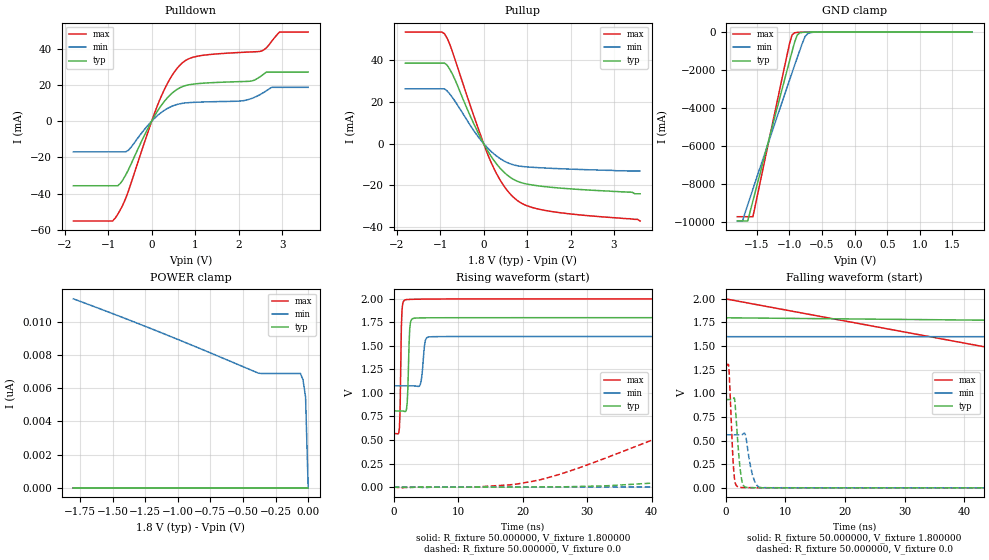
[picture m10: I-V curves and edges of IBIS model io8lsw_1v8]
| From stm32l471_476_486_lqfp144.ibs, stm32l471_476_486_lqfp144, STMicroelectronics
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|   Model io8lsw_1v8
[Model]  io8lsw_1v8
Model_type I/O
Polarity   Non-Inverting
Enable   Active-Low
Vinl =   0.540000V
Vinh =   1.260000V
Vmeas =  0.900000V
Cref =   100.000000nF
Rref =   1.000000k
Vref =   1.800000V
C_comp   3.002600pF   2.845500pF   3.023700pF
[Temperature Range]   25.000000   0.125000k   -40.000000
[Pullup Reference]   1.800000V   1.600000V   2.000000V
[Pulldown Reference]   0.0V   0.0V   0.0V
[POWER Clamp Reference]   1.800000V   1.600000V   2.000000V
[GND Clamp Reference]   0.0V   0.0V   0.0V
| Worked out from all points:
|   slope of the pulldown table from 0 to 0.27 V, typ, clamps not added: 26.4 ohm
|   slope of the pullup table from 0 to 0.27 V, typ, clamps not added: 30.1 ohm
|   GND clamp passes 1 mA (typ) near -0.58 V on its own axis
|   rising waveform, R_fixture 50.000000, V_fixture 1.800000: 20-80 % time 262ps typ, 404ps min, 194ps max; typ from 0.809 V to 1.8 V
|   rising waveform, R_fixture 50.000000, V_fixture 0.0: 20-80 % time 64.5ns typ, 115ns min, 35.9ns max; typ from 0 V to 0.934 V
|   falling waveform, R_fixture 50.000000, V_fixture 1.800000: 20-80 % time 75.9ns typ, 121ns min, 63ns max; typ from 1.8 V to 0.809 V
|   falling waveform, R_fixture 50.000000, V_fixture 0.0: 20-80 % time 713ps typ, 1.02ns min, 552ps max; typ from 0.934 V to 0 V
[Pulldown]
|Voltage   I(typ)   I(min)   I(max)
-1.8V     -35.64mA   -16.93mA   -55.1mA
-840mV    -35.64mA   -16.93mA   -53.52mA
-720mV    -34.31mA   -16.93mA   -48.86mA
-540mV    -27.04mA   -16.13mA   -38.89mA
240mV     9.303mA    5.14mA     14.78mA
480mV     15.67mA    8.374mA    25.64mA
720mV     19.18mA    9.883mA    32.46mA
1.08V     20.76mA    10.49mA    35.96mA
2.1V      21.86mA    11.27mA    37.98mA
2.52V     24.95mA    15.02mA    38.63mA
2.94V     27.08mA    18.65mA    49.17mA
3.6V      27.08mA    18.65mA    49.17mA
[Pullup]
|Voltage   I(typ)   I(min)   I(max)
-1.8V     38.39mA    26.12mA    53.23mA
-960mV    38.39mA    26.12mA    53.23mA
-900mV    38.39mA    26.12mA    52.4mA
-840mV    37.45mA    25.13mA    50.31mA
-720mV    33.22mA    22.05mA    44.01mA
-240mV    10.08mA    6.588mA    14.1mA
120mV     -4.38mA    -2.702mA   -6.45mA
420mV     -12.68mA   -7.723mA   -18.77mA
720mV     -17.48mA   -10.37mA   -26.28mA
1.02V     -19.45mA   -11.2mA    -29.89mA
1.44V     -20.66mA   -11.73mA   -32.03mA
3.6V      -24mA      -13.1mA    -37mA
[GND_clamp]
|Voltage   I(typ)   I(min)   I(max)
-1.8V     -9.93A     -9.932A    -9.707A
-1.72V    -9.93A     -9.932A    -9.707A
-1.64V    -9.93A     -9.083A    -9.707A
-1.56V    -8.876A    -8.251A    -9.707A
-1V       -1.54A     -2.541A    -631mA
-960mV    -1.028A    -2.139A    -153.7mA
-920mV    -527mA     -1.74A     -39.12mA
-880mV    -155.6mA   -1.344A    -18.01mA
-840mV    -45.32mA   -953mA     -12.68mA
-760mV    -8.418mA   -235mA     -7.62mA
-680mV    -3.44mA    -33.01mA   -3.865mA
1.8V      0A         0A         0A
[POWER_clamp]
|Voltage   I(typ)   I(min)   I(max)
-1.8V     0A         11.37nA    0A
-1.14V    0A         9.374nA    0A
-380mV    0A         6.895nA    0A
-60mV     0A         6.881nA    0A
-40mV     0A         6.518nA    0A
-20mV     0A         5.452nA    0A
0V        0A         0A         0A
[Ramp]
| variable   typ   min   max
dV/dt_r  0.56065/64.46590n   0.33678/0.11506u   0.77868/35.83006n
dV/dt_f  0.59454/66.72156n   0.31098/0.11332u   0.85907/35.23271n
R_load = 50.000000
[Rising Waveform]
R_fixture= 50.000000
V_fixture= 1.800000
V_fixture_min= 1.600000
V_fixture_max= 2.000000
|time   V(typ)   V(min)   V(max)
0s        808.7mV    1.076V     568.3mV
900.9ps   808.8mV    1.076V     631mV
1.301ns   808.5mV    1.076V     1.883V
1.802ns   801.7mV    1.076V     1.989V
2.102ns   893.2mV    1.076V     1.993V
2.503ns   1.684V     1.076V     1.994V
3.103ns   1.793V     1.075V     1.996V
4.204ns   1.798V     1.106V     1.997V
5.506ns   1.799V     1.595V     1.998V
49.85ns   1.8V       1.6V       2V
[Rising Waveform]
R_fixture= 50.000000
V_fixture= 0.0
V_fixture_min= 0.0
V_fixture_max= 0.0
|time   V(typ)   V(min)   V(max)
0s        812.2nV    1.073uV    103.9nV
13.21ns   -64.25uV   -37.99uV   2.552mV
22.82ns   1.132mV    -19.01uV   79.33mV
52.85ns   143.6mV    5.762mV    806.2mV
70.87ns   334.6mV    25mV       1.088V
104.5ns   645.3mV    117.3mV    1.258V
134.5ns   801.4mV    225.8mV    1.286V
167ns     878.7mV    332.9mV    1.295V
257.1ns   929.8mV    500.5mV    1.298V
598.2ns   934.4mV    561.5mV    1.298V
[Falling Waveform]
R_fixture= 50.000000
V_fixture= 1.800000
V_fixture_min= 1.600000
V_fixture_max= 2.000000
|time   V(typ)   V(min)   V(max)
0s        1.8V       1.6V       2V
50.05ns   1.77V      1.6V       1.414V
100.1ns   1.342V     1.568V     665.7mV
150.2ns   974.3mV    1.436V     591.4mV
200.2ns   869.8mV    1.276V     574.4mV
250.2ns   833.2mV    1.178V     570.2mV
300.3ns   819.1mV    1.134V     568.6mV
400.4ns   810.6mV    1.095V     568.3mV
550.6ns   808.9mV    1.079V     568.3mV
4.955us   808.7mV    1.076V     568.3mV
[Falling Waveform]
R_fixture= 50.000000
V_fixture= 0.0
V_fixture_min= 0.0
V_fixture_max= 0.0
|time   V(typ)   V(min)   V(max)
0s        934.4mV    561.5mV    1.298V
600.6ps   934.4mV    561.5mV    1.231V
1.201ns   937.7mV    561.5mV    360.7mV
1.502ns   944.6mV    561.5mV    97.21mV
2.102ns   442.2mV    561.2mV    9.829mV
2.603ns   126.4mV    561.1mV    4.131mV
3.003ns   23.99mV    572.4mV    2.988mV
4.505ns   1.417mV    139.8mV    1.9mV
5.806ns   916.8uV    4.324mV    1.584mV
49.85ns   812.2nV    1.073uV    103.9nV
